FUNCTION_BLOCK FB_CylinderDiag EXTENDS FB_Cylinder
(* FB_CylinderDiag	- number of control signals
							one direction is controllable
					- type of feedback signal
							feedback in base and work position
					- with diagnosis									*)
VAR_INPUT
	tiTimeOut 	 	: TIME;
END_VAR
VAR_OUTPUT
	bError			: BOOL;
	sErrorMsg		: STRING;
END_VAR
VAR
	rtrigError		: R_TRIG;
	bErrorMove		: BOOL;
	WatchDogTimer	: TON;
END_VAR

// =========================================================
;
// =========================================================

METHOD M_Diag : BOOL
VAR_INPUT
END_VAR
// =========================================================
	// Timer starts when cylinder is not in base and work position
	
IF NOT bAtBasePos AND NOT bAtWorkPos THEN
	WatchDogTimer(IN := TRUE, PT := tiTimeOut);
ELSE
	WatchDogTimer(IN := FALSE, PT := tiTimeOut);
END_IF

// =========================================================
	// Error if cylinder does not reach base or work position
	
rtrigError( CLK := WatchDogTimer.Q );
bError := WatchDogTimer.Q;

IF rtrigError.Q THEN
	bErrorMove := bMoveToWork;
END_IF

IF bError THEN
	IF bErrorMove = bMoveToWork THEN
		IF bMoveToWork THEN
			sErrorMsg := 'Work position not reached';
		ELSE
			sErrorMsg := 'Base position not reached';
		END_IF
	ELSE
		bError := FALSE;
		sErrorMsg := '';
	END_IF
ELSE
	sErrorMsg := '';
END_IF

// =========================================================
	// Return
	
M_Diag := bError;

// =========================================================
END_METHOD

METHOD PUBLIC M_Reset
VAR_INPUT
END_VAR
// =========================================================
	// Reset
	
SUPER^.M_Reset();		// Calling method M_Reset of base class FB_Cylinder via 'SUPER^.'
bError := FALSE;
sErrorMsg := '';

// =========================================================
END_METHOD

METHOD M_StateMachine : BOOL
VAR_INPUT
	bBasePosReq		: BOOL;
	bWorkPosReq		: BOOL;
END_VAR
// =========================================================
	// Call the method M_StateMachine of base class FB_Cylinder via 'SUPER^.'

SUPER^.M_StateMachine(	bBasePosReq := bBasePosReq,
						bWorkPosReq	:= bWorkPosReq );

// =========================================================
	// Additional diagnosis

M_StateMachine := M_Diag();

// =========================================================
END_METHOD

END_FUNCTION_BLOCK
